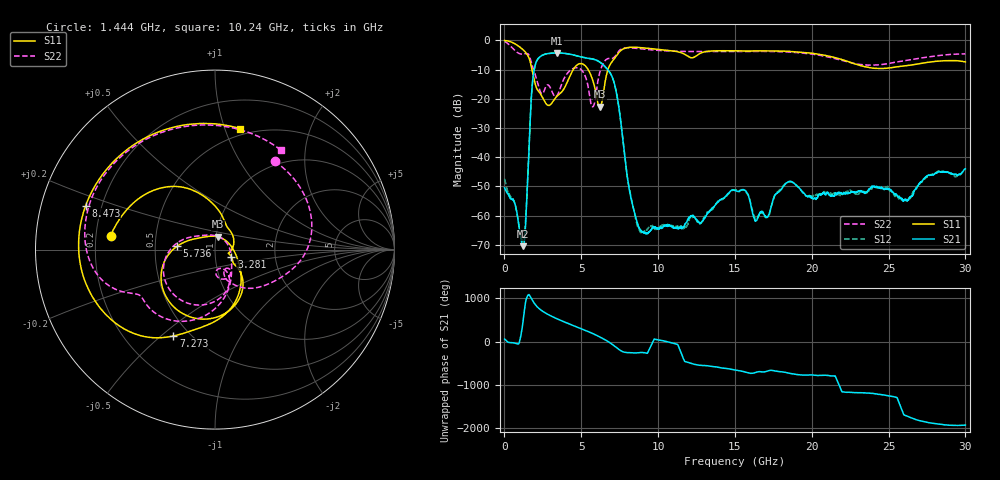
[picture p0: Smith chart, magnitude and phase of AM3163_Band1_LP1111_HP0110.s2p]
!Agilent Technologies,E8364B,MY43040894,A.07.50.67
!Agilent E8364B: A.07.50.67
!Date: Thursday, August 20, 2020 11:57:58
!Correction: S11(Full 2 Port(1,2))
!S21(Full 2 Port(1,2))
!S12(Full 2 Port(1,2))
!S22(Full 2 Port(1,2))
!S2P File: Measurements: S11, S21, S12, S22:
# Hz S  dB  R 50
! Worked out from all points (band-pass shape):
!   3201 points, 10 MHz to 30 GHz, reference 50 ohm
!   highest |S21| = -4.34 dB at 3.431 GHz (marker M1); lowest = -70.4 dB at 1.228 GHz (marker M2)
!   |S21| within 3 dB of the highest: 2.072 GHz to 6.181 GHz (4.109 GHz wide, 99.6 % of centre)
!   lowest |S11| = -22.7 dB at 6.195 GHz (marker M3), VSWR 1.16, Z = 51 + j7.34 ohm
!   |S11| at or under -10 dB: 1.787 GHz to 4.478 GHz (2.691 GHz wide, 85.9 % of centre); 5.444 GHz to 6.738 GHz (1.294 GHz wide, 21.2 % of centre)
!   |S22| runs from -22.7 to -0.4 dB; largest |S21 - S12| = 0.0048
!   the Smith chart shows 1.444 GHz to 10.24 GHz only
!   S11 on the Smith chart (normalised r, x): 1.444 GHz: 0.26, +0.06; 3.281 GHz: 1.20, -0.10; 5.736 GHz: 0.65, +0.03; 7.273 GHz: 0.41, -0.55; 8.473 GHz: 0.14, +0.16; 10.24 GHz: 0.44, +1.13
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1e7  -0.05 -8.0  -50.48 58.7  -47.38 -12.3  -0.40 -14.9
7.316344e8  -1.34 -87.9  -57.03 -43.1  -57.10 -42.1  -3.72 -148.5
1.228344e9  -3.31 -152.9  -70.44 163.1  -68.89 -85.8  -4.68 107.4
1.443897e9  -4.63 172.3  -55.76 -73.9  -55.02 1.9  -4.52 55.9
1.95935e9  -13.98 80.0  -9.46 159.1  -9.47 159.0  -10.97 -49.6
2.474803e9  -19.55 12.6  -5.08 -13.8  -5.09 -13.8  -18.28 -58.6
3.280784e9  -19.98 -23.8  -4.36 -168.7  -4.37 -168.7  -19.22 -80.7
3.430734e9  -19.07 -29.8  -4.34 167.2  -4.35 167.2  -18.89 -69.2
4.021162e9  -15.06 -40.2  -4.54 77.7  -4.56 77.7  -11.81 -79.6
5.014581e9  -7.99 -118.2  -5.73 -63.9  -5.72 -63.6  -10.15 -157.7
5.736216e9  -13.49 174.8  -6.41 -171.0  -6.38 -171.1  -22.74 55.1
6.195438e9  -22.72 77.8  -7.39 109.8  -7.43 109.7  -11.17 -79.8
7.273203e9  -5.45 -115.7  -17.55 -134.8  -17.55 -134.2  -4.95 -155.5
8.472803e9  -2.37 161.2  -59.15 97.3  -59.42 101.7  -2.69 131.4
1.000979e10  -3.12 88.3  -64.31 39.5  -64.37 42.0  -3.45 65.6
1.024409e10  -3.24 78.3  -64.04 26.0  -63.23 22.6  -3.53 56.6
1.5005e10  -3.59 -71.9  -51.40 61.1  -51.23 63.3  -3.79 -92.5
1.634518e10  -3.63 -104.3  -61.70 6.9  -61.08 8.8  -3.79 -125.2
2.000958e10  -4.41 162.8  -53.91 -52.4  -53.64 -52.7  -4.71 135.5
2.274617e10  -7.98 59.8  -51.82 -97.6  -52.14 -97.4  -7.93 20.2
2.500479e10  -9.51 -62.9  -50.88 -174.1  -50.74 -169.0  -7.96 -93.1
3e10  -7.39 104.6  -43.94 -132.2  -44.72 -140.5  -4.64 100.3
